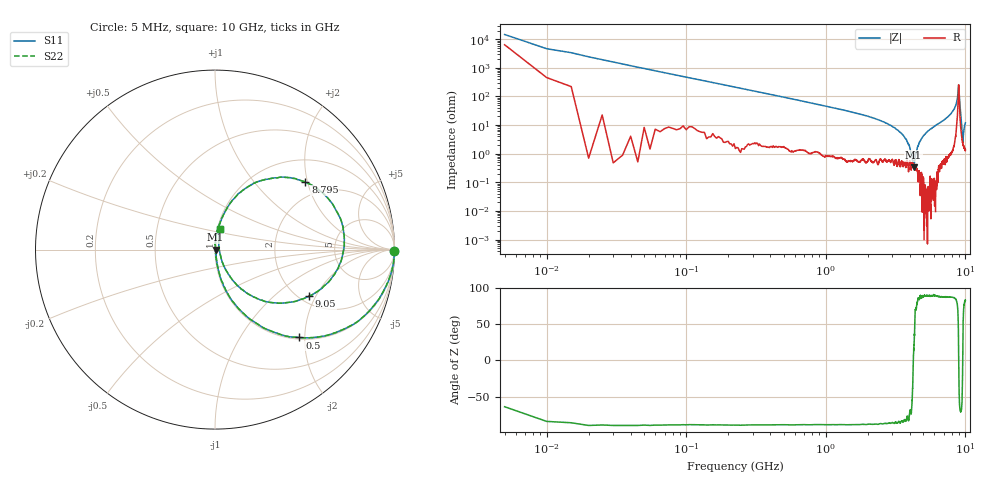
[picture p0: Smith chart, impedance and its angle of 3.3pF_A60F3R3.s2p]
! Amotech Co.,Ltd.
! http://www.amotech.co.kr/
! Part Number: A60F3R3
! These Parameters are Measured in Series Mode Connection
! Operation Temp=25[degC], DC Bias Voltage=0[V]
! Freq. Start=5[MHz] Stop=10[GHz], 2000[Steps]
! Date: Monday, July 20, 2020, 03:59:30
# GHZ S RI R 50.000000
!Freq.(Hz) S11(Real) S11(Imag) S21(Real) S21(Imag) S12(Real) S12(Imag) S22(Real) S22(Imag)
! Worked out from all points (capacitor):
!   2000 points, 5 MHz to 10 GHz, reference 50 ohm
!   read as one part in series: C = 3.37 pF near 55 MHz
!   lowest |Z| = 332 mohm at 4.25 GHz (marker M1)
!   series resonance near 4.233 GHz, so ESL is about 420 pH
!   S11 on the Smith chart (normalised r, x): 5 MHz: open; 500 MHz: 1.04, -1.88; 8.795 GHz: 1.56, +1.94; 9.05 GHz: 2.23, -1.76; 10 GHz: 1.03, +0.24
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0.005  0.997 -0.00611  0.00302 0.00611  0.00302 0.00611  0.997 -0.00611
0.065  0.9804 -0.1348  0.0196 0.1348  0.0196 0.1348  0.9804 -0.1348
0.135  0.9221 -0.2603  0.0779 0.2603  0.0779 0.2603  0.9221 -0.2603
0.28  0.7395 -0.4324  0.2605 0.4324  0.2605 0.4324  0.7395 -0.4324
0.5  0.4702 -0.4897  0.5298 0.4897  0.5298 0.4897  0.4702 -0.4897
0.945  0.1958 -0.388  0.8042 0.388  0.8042 0.388  0.1958 -0.388
1.675  0.0668 -0.2387  0.9332 0.2387  0.9332 0.2387  0.0668 -0.2387
3.34  0.00986 -0.0599  0.9901 0.0599  0.9901 0.0599  0.00986 -0.0599
3.955  0.00435 -0.0191  0.9956 0.0191  0.9956 0.0191  0.00435 -0.0191
4.25  0.00327 0.000496  0.9967 -0.000496  0.9967 -0.000496  0.00327 0.000496
4.555  0.00246 0.0176  0.9975 -0.0176  0.9975 -0.0176  0.00246 0.0176
5.005  0.00322 0.0419  0.9968 -0.0419  0.9968 -0.0419  0.00322 0.0419
6.67  0.0202 0.1246  0.9798 -0.1246  0.9798 -0.1246  0.0202 0.1246
8.335  0.1373 0.3168  0.8627 -0.3168  0.8627 -0.3168  0.1373 0.3168
8.6  0.259 0.3846  0.741 -0.3846  0.741 -0.3846  0.259 0.3846
8.795  0.504 0.3768  0.496 -0.3768  0.496 -0.3768  0.504 0.3768
8.945  0.7201 0.0378  0.2799 -0.0378  0.2799 -0.0378  0.7201 0.0378
9.05  0.5229 -0.2603  0.4771 0.2603  0.4771 0.2603  0.5229 -0.2603
9.245  0.13 -0.2039  0.87 0.2039  0.87 0.2039  0.13 -0.2039
9.565  0.0233 0.000603  0.9767 -0.000603  0.9767 -0.000603  0.0233 0.000603
9.795  0.0215 0.0719  0.9785 -0.0719  0.9785 -0.0719  0.0215 0.0719
10  0.0273 0.1151  0.9727 -0.1151  0.9727 -0.1151  0.0273 0.1151
